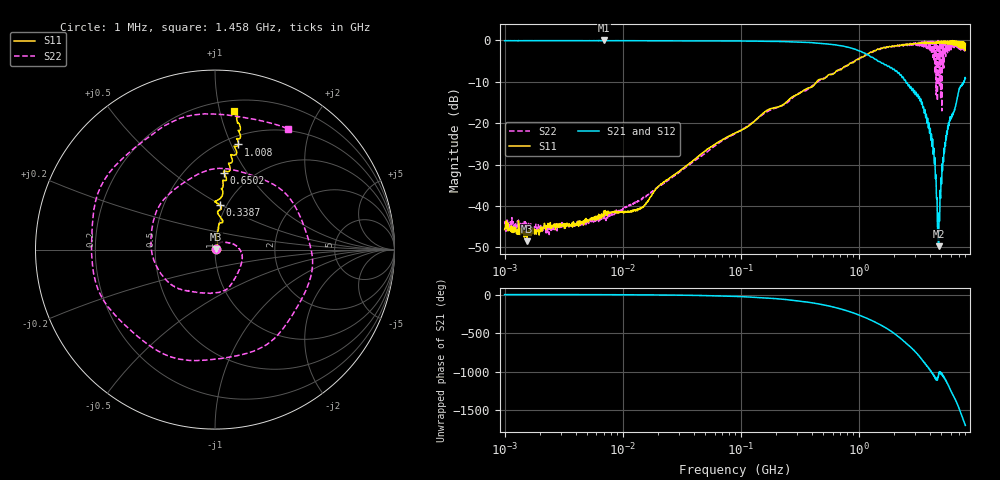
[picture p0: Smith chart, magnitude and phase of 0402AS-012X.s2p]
!s-Parameter Generated by FASTRON Sdn. Bhd.
!FASTRON P/N : 0402AS-012X
!Keysight Technologies: E5071C_MY46733604_B.14.02
!Date: Mon Dec 01 10:30:46 2025
!Version  :Rev00  Mon Dec 01 10:30:46 2025
!Data & Calibration Information:
!Freq  S11:SOLT2(ON)  S21:SOLT2(ON)  S12:SOLT2(ON)  S22:SOLT2(ON)
!PortZ  Port1:50+j0  Port2:50+j0
!When reading reference impedance value at option line is always used.
! Remarks : This data is being provided solely for informational purposes.
# Hz S dB R 50
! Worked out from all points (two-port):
!   1601 points, 1 MHz to 8 GHz, reference 50 ohm
!   highest |S21| = 0.00 dB at 6.912 MHz (marker M1); lowest = -49.7 dB at 4.745 GHz (marker M2)
!   |S21| within 3 dB of the highest: start of sweep to 1.111 GHz
!   lowest |S11| = -48.5 dB at 1.541 MHz (marker M3), VSWR 1.01, Z = 50.4 + j0.131 ohm
!   |S11| at or under -10 dB: start of sweep to 439.1 MHz
!   |S22| runs from -46.9 to 0.0 dB; largest |S21 - S12| = 0.021
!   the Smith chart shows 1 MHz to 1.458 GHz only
!   S11 on the Smith chart (normalised r, x): 1 MHz: 1.01, +0.00; 338.7 MHz: 0.93, +0.49; 650.2 MHz: 0.75, +0.79; 1.008 GHz: 0.58, +1.06; 1.458 GHz: 0.28, +1.11
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1000000  -45.70 15.4  -0.07 -0.3  -0.04 -0.3  -43.70 12.8
1541011  -48.50 20.2  -0.06 -0.4  -0.05 -0.5  -45.20 -1.2
4479405  -43.80 35.9  -0.06 -1.3  -0.05 -1.2  -44.30 39.3
6911657  -41.20 31.9  0.00 -2.0  -0.11 -1.7  -41.40 36.6
2.00676e7  -35.30 58.9  -0.06 -5.6  -0.06 -5.5  -35.40 65.3
8.994653e7  -22.30 85.5  -0.12 -24.5  -0.12 -24.5  -22.50 31.8
3.386818e8  -12.10 83.3  -0.43 -90.8  -0.42 -90.8  -12.30 -89.9
4.006501e8  -11.20 87.3  -0.53 -107.0  -0.53 -107.0  -11.00 -126.0
6.502164e8  -7.30 83.4  -1.12 -173.0  -1.11 -173.0  -7.56 109.0
1.007883e9  -4.44 77.5  -2.50 93.1  -2.49 93.0  -4.37 -72.7
1.233539e9  -2.93 79.1  -3.72 35.4  -3.72 35.3  -3.14 169.0
1.457824e9  -2.14 82.1  -5.04 -18.1  -5.03 -18.2  -2.09 59.0
1.7949e9  -1.57 88.3  -6.19 -97.1  -6.20 -97.2  -1.67 -105.0
2.114474e9  -1.19 94.2  -7.56 -176.0  -7.55 -176.0  -1.33 92.2
2.472225e9  -1.10 98.8  -9.53 99.2  -9.51 99.1  -1.24 -82.6
2.853703e9  -0.92 107.0  -11.70 14.3  -11.70 14.0  -0.96 98.1
3.203473e9  -0.66 115.0  -14.00 -69.2  -14.00 -69.5  -0.49 -79.7
3.568312e9  -0.40 127.0  -17.10 -163.0  -17.00 -164.0  -1.06 76.2
3.933151e9  -0.67 130.0  -19.90 118.0  -19.90 117.0  -1.85 -78.3
4.296652e9  -0.61 138.0  -26.70 42.8  -26.80 42.3  -0.26 115.0
4.744521e9  -0.23 146.0  -49.70 43.3  -49.60 43.3  -10.80 122.0
8e9  -0.71 -103.0  -9.14 99.3  -9.17 98.9  -2.44 134.0
